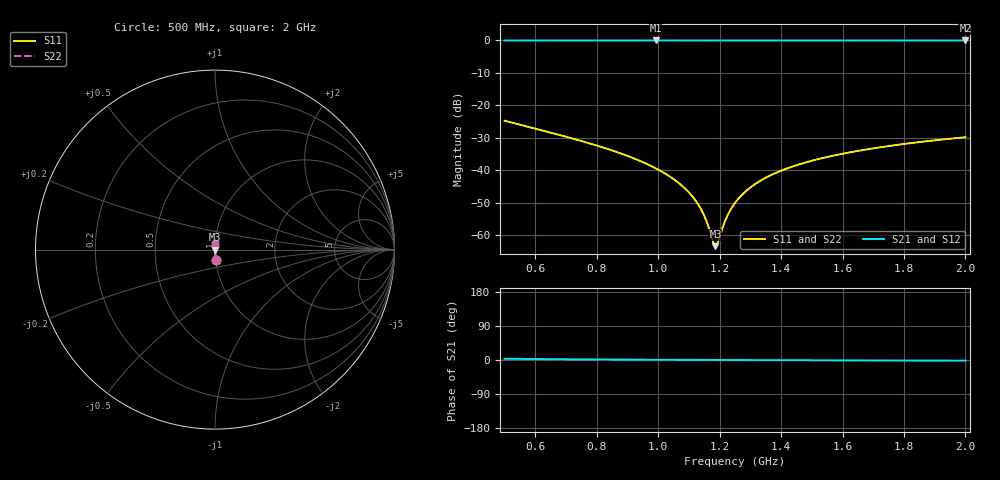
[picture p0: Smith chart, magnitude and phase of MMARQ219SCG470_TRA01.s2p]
! MMARQ219SCG470_TRA01  S-PARAMETER MODEL  ( General Type )
! Model Generated by TAIYO YUDEN Corporation (http://www.ty-top.com)
! Version 1.0
! TAIYO YUDEN Control No. 150609
! Copyright(c) 2015 TAIYO YUDEN CO.,LTD. All Rights Reserved.
! Product Description (link to TY-COMPAS)
! https://ds.yuden.co.jp/TYCOMPAS/or/detail?pn=MMARQ219SCG470JTRA01&u=M
! Products Name : Multilayer Ceramic Capacitors
! Characteristics :
!  Capacitance : 47 pF , Rated Voltage : 250V , TCC : CG / C0G
!  Case Size : 2.0 x 1.25 / 0.079 x 0.049 [mm/inch] , Thickness : 0.85 / 0.033 [mm/inch]
!  (Conditions: Temperature = 25 degC , DC Bias Current/Voltage = 0A / 0V)
! External Node Assignments :
!  1  o---| |---o  2
! GND o---------o GND
! Frequency Range : 500MHz  -  2GHz  [ 401 STEP ]
# MHz S RI R 50
! Freq[MHz].  S11 Real  S11 Imag  S21 Real  S21 Imag  S12 Real  S12 Imag  S22 Real  S22 Imag
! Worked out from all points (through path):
!   401 points, 500 MHz to 2 GHz, reference 50 ohm
!   highest |S21| = -0.01 dB at 991.2 MHz (marker M1); lowest = 0.0 dB at 2 GHz (marker M2)
!   lowest |S11| = -63.3 dB at 1.186 GHz (marker M3), VSWR 1.00, Z = 50.1 - j0.00473 ohm
!   |S11| at or under -10 dB: start of sweep to end of sweep
!   |S22| runs from -63.3 to -24.7 dB; largest |S21 - S12| = 0
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500  0.00372 -0.0581  0.9963 0.0581  0.9963 0.0581  0.00372 -0.0581
751.25  0.0012 -0.0282  0.9988 0.0282  0.9988 0.0282  0.0012 -0.0282
890  0.00078 -0.0174  0.9992 0.0174  0.9992 0.0174  0.00078 -0.0174
991.25  0.000656 -0.0108  0.9993 0.0108  0.9993 0.0108  0.000656 -0.0108
1002.5  0.000649 -0.0101  0.9994 0.0101  0.9994 0.0101  0.000649 -0.0101
1070  0.000632 -0.00621  0.9994 0.00621  0.9994 0.00621  0.000632 -0.00621
1118.75  0.000643 -0.00354  0.9994 0.00354  0.9994 0.00354  0.000643 -0.00354
1133.75  0.000649 -0.00275  0.9994 0.00275  0.9994 0.00275  0.000649 -0.00275
1148.75  0.000657 -0.00196  0.9993 0.00196  0.9993 0.00196  0.000657 -0.00196
1160  0.000664 -0.00138  0.9993 0.00138  0.9993 0.00138  0.000664 -0.00138
1178.75  0.000677 -0.000425  0.9993 0.000425  0.9993 0.000425  0.000677 -0.000425
1186.25  0.000683 -4.72e-05  0.9993 4.72e-05  0.9993 4.72e-05  0.000683 -4.72e-05
1193.75  0.00069 0.000329  0.9993 -0.000329  0.9993 -0.000329  0.00069 0.000329
1223.75  0.000718 0.00181  0.9993 -0.00181  0.9993 -0.00181  0.000718 0.00181
1250  0.000746 0.00307  0.9993 -0.00307  0.9993 -0.00307  0.000746 0.00307
1291.25  0.000798 0.00501  0.9992 -0.00501  0.9992 -0.00501  0.000798 0.00501
1343.75  0.000876 0.0074  0.9991 -0.0074  0.9991 -0.0074  0.000876 0.0074
1415  0.001 0.0105  0.999 -0.0105  0.999 -0.0105  0.001 0.0105
1501.25  0.00118 0.0141  0.9988 -0.0141  0.9988 -0.0141  0.00118 0.0141
1613.75  0.00144 0.0186  0.9986 -0.0186  0.9986 -0.0186  0.00144 0.0186
1752.5  0.00183 0.0238  0.9982 -0.0238  0.9982 -0.0238  0.00183 0.0238
2000  0.00264 0.0324  0.9974 -0.0324  0.9974 -0.0324  0.00264 0.0324
